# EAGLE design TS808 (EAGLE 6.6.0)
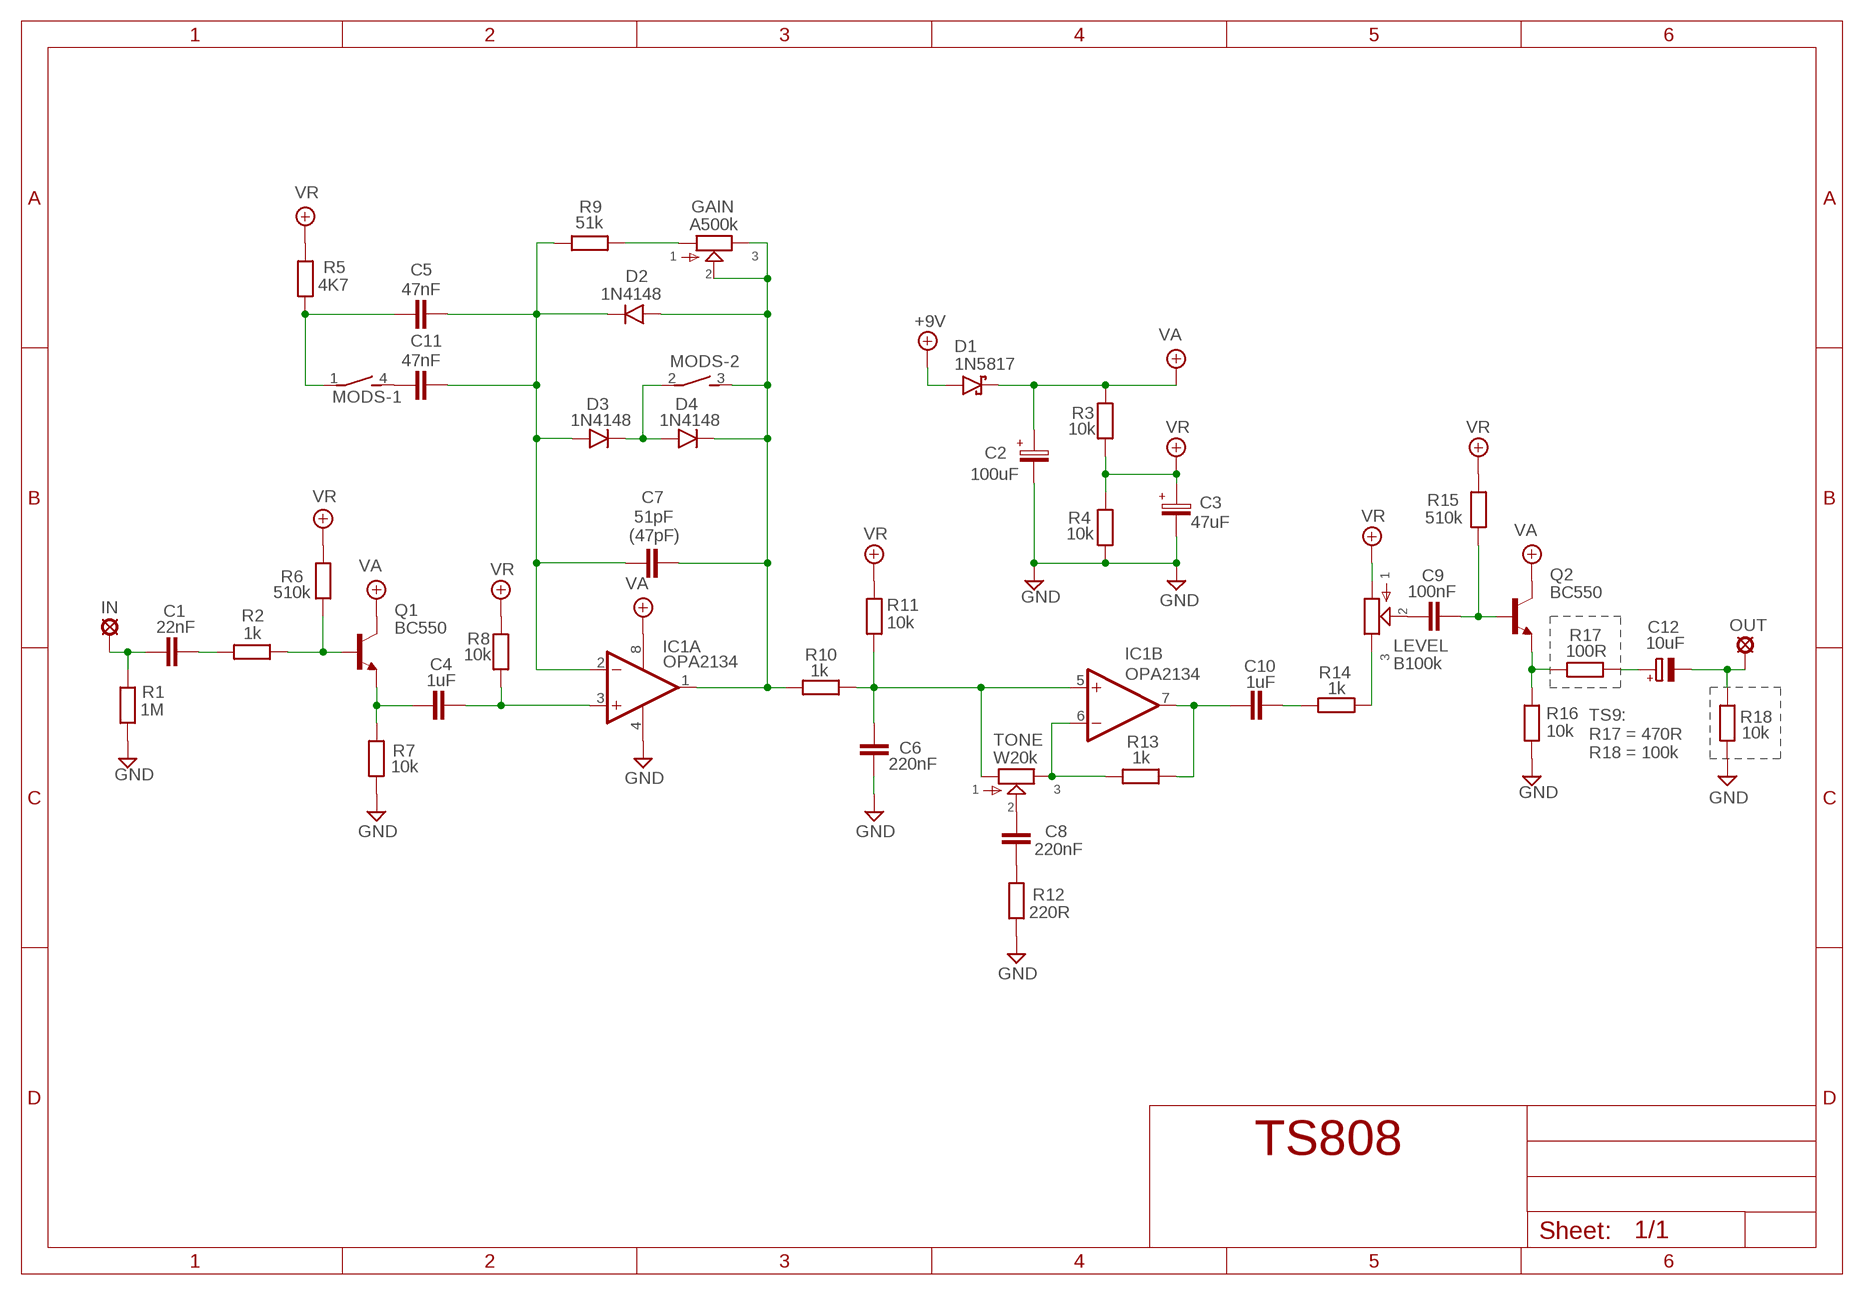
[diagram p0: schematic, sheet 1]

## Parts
+9V  +9V  +9V(T)1  [ROUND]
C1  22nF  22NF-82NF"  [4,5MM]
C2  100uF  063-EU  [063_025]
C3  47uF  063-EU  [063_025]
C4  1uF  072X0352  [072X035]
C5  47nF  22NF-82NF"  [4,5MM]
C6  220nF  100NF-220NF  [7,5MM]
C7  51pF  050X030_0251  [050X030_025]
C8  220nF  100NF-220NF  [7,5MM]
C9  100nF  100NF-220NF  [7,5MM]
C10  1uF  072X0352  [072X035]
C11  47nF  22NF-82NF"  [4,5MM]
C12  10uF  CPOL-EUE5-4  [E5-4]
D1  1N5817  [DO41-3]
D2  1N4148  1N4148-3  [DO35-3]
D3  1N4148  1N4148-3  [DO35-3]
D4  1N4148  1N4148-3  [DO35-3]
GAIN  A500k  POT-EU16MM  [16MM]
GND  GND  GND(T)1  [ROUND]
GND1  GND  GND(T)1  [ROUND]
IC1  OPA2134  LM4558N  [DIL08]
IN  MCS10B  [MCS10B]
LEVEL  B100k  POT-EU16MM  [16MM]
MODS  DS02E  [DS-02]
OUT  MCS10B  [MCS10B]
Q1  BC550  [TO92-]
Q2  BC550  [TO92-]
R1  1M  6MM-EU3  [R0207/3]
R2  1k  6MM-EU3  [R0207/3]
R3  10k  6MM-EU3  [R0207/3]
R4  10k  6MM-EU3  [R0207/3]
R5  4K7  6MM-EU3  [R0207/3]
R6  510k  6MM-EU3  [R0207/3]
R7  10k  6MM-EU3  [R0207/3]
R8  10k  6MM-EU3  [R0207/3]
R9  51k  6MM-EU3  [R0207/3]
R10  1k  6MM-EU3  [R0207/3]
R11  10k  6MM-EU3  [R0207/3]
R12  220R  6MM-EU3  [R0207/3]
R13  1k  6MM-EU3  [R0207/3]
R14  1k  6MM-EU3  [R0207/3]
R15  510k  6MM-EU3  [R0207/3]
R16  10k  6MM-EU3  [R0207/3]
R17  100R  6MM-EU3  [R0207/3]
R18  10k  6MM-EU3  [R0207/3]
TONE  W20k  POT-EU16MM  [16MM]

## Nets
+9V: +9V.1(+9V) D1.A
GND: C2.- C3.- C6.P$2 GND1.1(GND) GND.1(GND) IC1.4(P:V-) R1.1 R4.1 R7.1 R12.1 R16.1 R18.1
N$1: C8.P$1 TONE.2
N$2: C1.2 R2.1
N$3: Q1.2(B) R2.2 R6.1
N$4: C4.2 IC1.3(A:+IN) R8.1
N$5: C5.2 C7.1 C11.2 D2.C D3.A IC1.2(A:-IN) R9.1
N$6: C4.1 Q1.1(E) R7.2
N$7: C8.P$2 R12.2
N$8: GAIN.1 R9.2
N$9: C9.P$1 LEVEL.2
N$10: IC1.6(B:-IN) R13.1 TONE.3
N$11: C6.P$1 IC1.5(B:+IN) R10.2 R11.1 TONE.1
N$12: C11.1 MODS.4
N$13: D3.C D4.A MODS.2
N$14: C10.1 IC1.7(B:OUT) R13.2
N$15: C10.2 R14.1
N$16: LEVEL.3 R14.2
N$17: Q2.1(E) R16.2 R17.1
N$18: C1.1 IN.MP R1.2
N$19: C9.P$2 Q2.2(B) R15.1
N$20: C12.+ R17.2
N$21: C12.- OUT.MP R18.2
N$22: C7.2 D2.A D4.C GAIN.2 GAIN.3 IC1.1(A:OUT) MODS.3 R10.1
N$23: C5.1 MODS.1 R5.1
VA: C2.+ D1.C IC1.8(P:V+) Q1.3(C) Q2.3(C) R3.2
VR: C3.+ LEVEL.1 R3.1 R4.2 R5.2 R6.2 R8.2 R11.2 R15.2

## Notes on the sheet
- (47pF)
- TS9:
  R17 = 470R
  R18 = 100k

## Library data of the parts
+9V = gm-supply:+9V(T): +9V Voltage Supply
C1 C5 C11 = Mylar Kondensaattorit:22NF-82NF: 22nF-82nF
C2 C3 = Elektrolyytit:063-EU
C4 C10 = Wima MKS:072X035: 0.15 - 1.0uF;
C6 C8 C9 = Mylar Kondensaattorit:100NF-220NF: 100nF-220nF
C7 = Keraamiset kondensaattorit:050X030_025: 47 - 120pF
C12 = rcl:CPOL-EU: POLARIZED CAPACITOR, European symbol
D1 = Diodit:1N5817
D2-D4 = Diodit:1N4148: Fast Switching Diode
GAIN LEVEL TONE = gm-pots:POT-EU
GND GND1 = gm-supply:GND(T): Ground
IC1 = Operaatiovahvistimet:*4558: *4558 Op Amp Infamous for its use in tube screamers. This op amp has many manufacturers, hence the leading "*" in the name. The JRC4558 is a widely used example.
IN OUT = Padit:MCS10B: SOLDER PAD
MODS = switch-dil:DS02E: DIL/CODE SWITCH; OC_FARNELL: 9472126; OC_NEWARK: unknown
Q1 Q2 = Transistorit:BC550
R1-R18 = Vastukset:6MM-EU: 6mm Resistors (European schematic symbol)

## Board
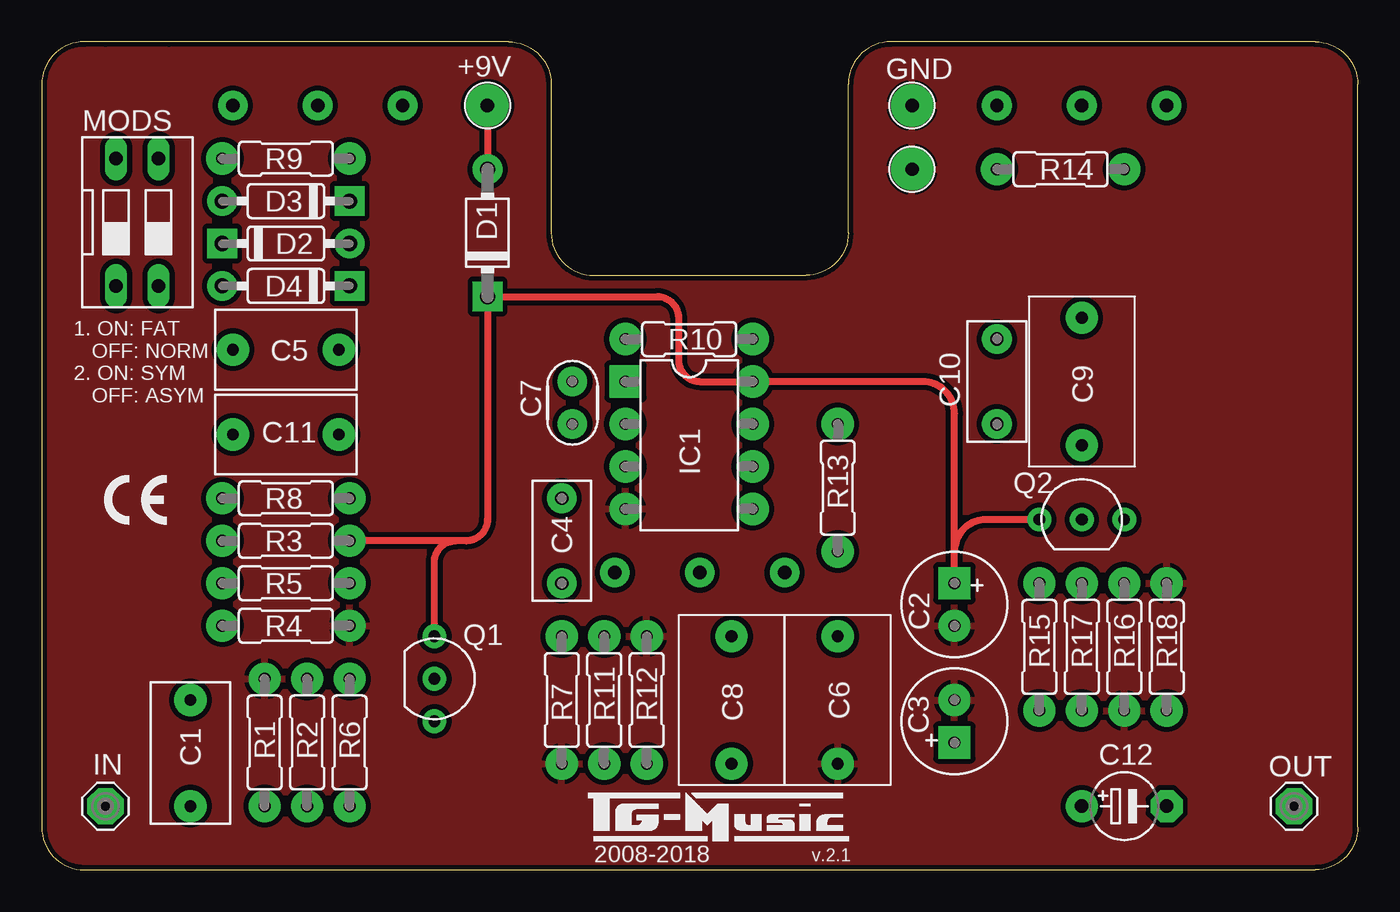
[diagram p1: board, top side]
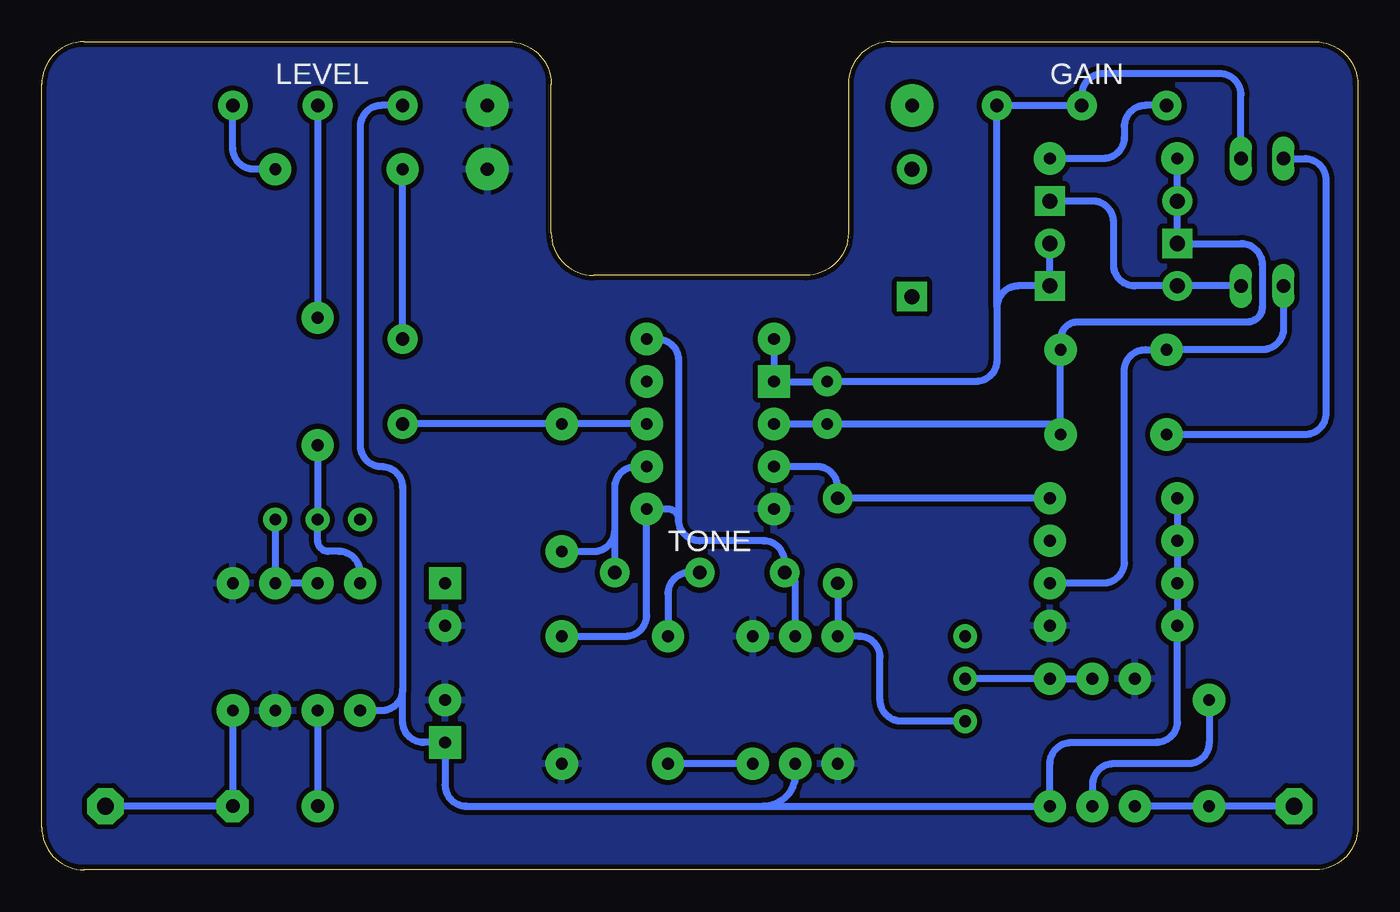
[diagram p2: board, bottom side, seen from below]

Size 78.74 x 49.53 mm. Coordinates in mm from the lower left corner, seen from the top.
Outline: 7.62,49.53 3.81,49.53
Outline: 78.74,2.54 78.74,46.99 arc90 76.2,49.53 50.8,49.53 arc90 48.26,46.99 48.26,38.1 arc-90 45.72,35.56 33.02,35.56 arc-90 30.48,38.1 30.48,46.99 arc90 27.94,49.53 2.54,49.53 arc90 0,46.99 0,2.54 arc90 2.54,0 76.2,0 arc90 78.74,2.54
Copper layers (1*16): Top 0.035mm / dielectric 1.5mm / Bottom 0.035mm
Design rules "ITEADstudio": minimum track width 10mil, minimum drill 12mil, track to track 12mil, track to pad 12mil, pad to pad 12mil, via to via 12mil, smd to smd 0mil, copper to edge 12mil, drill to drill 12mil, minimum pad ring 10mil, minimum via ring 6mil, stop-mask expansion 4mil, vias tented up to drill 100mil, thermal gap 10mil

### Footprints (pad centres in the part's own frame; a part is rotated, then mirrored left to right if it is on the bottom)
ROUND = drill 0.8 pad 2.54: 1 0,0
4,5MM = drill 0.7 pad 1.93: 1 -3.175,0; 2 3.175,0
063_025 = drill 0.7 pad 1.93 square: + -1.27,0 | drill 0.7 pad 1.93: - 1.27,0
072X035 = drill 0.8 pad 1.778: 1 -2.54,0; 2 2.54,0
7,5MM = drill 0.7 pad 1.93: P$1 -3.81,0; P$2 3.81,0
050X030_025 = drill 0.7 pad 1.778: 1 -1.27,0; 2 1.27,0
E5-4 = drill 0.813 pad 1.905: + -2.54,0 | drill 0.813 pad 1.905 octagon: - 2.54,0
DO41-3 = drill 0.9 pad 1.778: A 3.81,0 | drill 0.9 pad 1.778 square: C -3.81,0
DO35-3 = drill 0.9 pad 1.778: A 3.81,0 | drill 0.9 pad 1.778 square: C -3.81,0
16MM = drill 0.8 pad 1.778: 1 5.08,0; 2 0,0; 3 -5.08,0
DIL08 = drill 0.7 pad 1.93 square: 1 -3.81,-3.81 | drill 0.7 pad 1.93: 2 -1.27,-3.81; 3 1.27,-3.81; 4 3.81,-3.81; 5 3.81,3.81; 6 1.27,3.81; 7 -1.27,3.81; 8 -3.81,3.81
MCS10B = drill 1.016 pad 2.159 octagon: MP 0,0
DS-02 = drill 0.813 long: 1 -1.27,-3.81; 2 1.27,-3.81; 3 1.27,3.81; 4 -1.27,3.81
TO92- = drill 0.7 pad 1.422: 1 2.54,0; 2 0,0; 3 -2.54,0
R0207/3 = drill 0.7 pad 1.93: 1 -3.81,0; 2 3.81,0

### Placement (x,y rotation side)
+9V  26.67,45.72 0 top
C1  8.89,6.99 90 top
C2  54.61,15.88 270 top
C3  54.61,8.89 90 top
C4  31.11,19.68 90 top
C5  14.61,31.11 0 top
C6  47.62,10.16 270 top
C7  31.75,27.94 90 top
C8  41.27,10.16 270 top
C9  62.23,29.21 270 top
C10  57.15,29.21 90 top
C11  14.61,26.04 0 top
C12  64.77,3.81 0 top
D1  26.67,38.1 90 top
D2  14.61,37.47 0 top
D3  14.61,40.01 180 top
D4  14.61,34.92 180 top
GAIN  16.51,45.72 0 bottom
GND  52.07,45.72 0 top
GND1  52.07,41.91 0 top
IC1  38.73,25.4 270 top
IN  3.81,3.81 0 top
LEVEL  62.23,45.72 0 bottom
MODS  5.71,38.73 0 top
OUT  74.93,3.81 0 top
Q1  23.5,11.43 270 top
Q2  62.23,20.95 0 top
R1  13.34,7.62 270 top
R2  15.88,7.62 90 top
R3  14.61,19.68 0 top
R4  14.61,14.61 180 top
R5  14.61,17.14 180 top
R6  18.41,7.62 270 top
R7  31.11,10.16 90 top
R8  14.61,22.23 180 top
R9  14.61,42.55 0 top
R10  38.73,31.75 0 top
R11  33.66,10.16 270 top
R12  36.2,10.16 270 top
R13  47.62,22.86 90 top
R14  60.96,41.91 0 top
R15  59.69,13.34 270 top
R16  64.77,13.34 90 top
R17  62.23,13.34 270 top
R18  67.31,13.34 270 top
TONE  39.37,17.78 0 bottom

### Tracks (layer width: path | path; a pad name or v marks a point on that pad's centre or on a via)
+9V
  Top 0.406: +9V.1 D1.A
GND
  pour Bottom: 0,2.54 0,46.99 arc-90 2.54,49.53 27.94,49.53 arc-90 30.48,46.99 30.48,38.1 arc90 33.02,35.56 45.72,35.56 arc90 48.26,38.1 48.26,46.99 arc-90 50.8,49.53 76.2,49.53 arc-90 78.74,46.99 78.74,1.91 arc-90 76.83,0 2.54,0 arc-90
  pour Top: 0,2.54 0,46.99 arc-90 2.54,49.53 27.94,49.53 arc-90 30.48,46.99 30.48,38.1 arc90 33.02,35.56 45.72,35.56 arc90 48.26,38.1 48.26,46.99 arc-90 50.8,49.53 75.56,49.53 arc-90 78.74,46.35 78.74,2.54 arc-90 76.2,0 2.54,0 arc-90
N$1
  Bottom 0.406: TONE.2 40.01,17.78 arc-90 41.27,16.51 C8.P$1
N$2
  Bottom 0.406: C1.2 8.89,7.62 arc90 10.16,6.35 14.61,6.35 arc-90 15.88,5.08 R2.1
N$3
  Bottom 0.406: R2.2 R6.1 Q1.2
N$4
  Bottom 0.406: IC1.3 32.38,24.13 arc90 31.11,22.86 C4.2 R8.1
N$5
  Bottom 0.406: R9.1 D3.A D2.C 6.99,37.47 arc90 5.71,36.2 5.71,33.66 arc90 6.6,32.77 16.76,32.77 arc-90 17.78,31.75 C5.2 C11.2 arc-90 18.41,26.67 C7.1 IC1.2
N$6
  Bottom 0.406: C4.1 R7.2 29.84,13.97 arc90 28.57,12.7 28.57,10.16 arc-90 27.3,8.89 Q1.1
N$7
  Bottom 0.406: R12.2 C8.P$2
N$8
  Bottom 0.406: GAIN.1 12.7,45.72 arc-90 13.97,44.45 13.97,43.81 arc90 15.24,42.55 R9.2
N$9
  Bottom 0.406: LEVEL.2 C9.P$1
N$10
  Bottom 0.406: TONE.3 44.45,20.32 | 44.45,20.32 44.45,22.86 arc90 43.18,24.13 IC1.6 | R13.1 45.72,19.05 arc-90 44.45,20.32
N$11
  Bottom 0.406: R10.2 41.91,31.75 arc90 40.64,30.48 40.64,20.95 | R11.1 33.66,17.14 arc-90 TONE.1 34.29,18.41 arc-90 35.56,19.68 39.37,19.68 arc90 40.64,20.95 | C6.P$1 43.81,13.97 arc-90 42.55,15.24 IC1.5 41.27,21.59 arc90 40.64,20.95
N$12
  Bottom 0.406: MODS.4 3.17,42.55 arc90 1.91,41.27 1.91,27.3 arc90 3.17,26.04 C11.1
N$13
  Bottom 0.406: MODS.2 D4.A 13.34,34.92 arc90 14.61,36.2 14.61,38.73 arc-90 15.88,40.01 D3.C
N$14
  Bottom 0.406: IC1.7 R13.2 C10.1
N$15
  Bottom 0.406: C10.2 R14.1
N$16
  Bottom 0.406: R14.2 66.04,41.91 arc90 67.31,43.18 LEVEL.3
N$17
  Bottom 0.406: Q2.1 R16.2 R17.1
N$18
  Bottom 0.406: IN.MP C1.1 R1.2
N$19
  Bottom 0.406: C9.P$2 Q2.2 62.23,19.68 arc-90 61.59,19.05 60.96,19.05 arc90 59.69,17.78 R15.1
N$20
  Bottom 0.406: R17.2 C12.+
N$21
  Bottom 0.406: R18.2 C12.- OUT.MP
N$22
  Bottom 0.406: MODS.3 6.99,46.35 arc-90 8.26,47.62 15.24,47.62 arc-90 16.51,46.35 GAIN.2 GAIN.3 21.59,33.66 | D2.A D4.C 20.32,34.92 arc-90 21.59,33.66 | R10.1 IC1.1 C7.2 22.86,29.21 arc-90 21.59,30.48 21.59,33.66
N$23
  Bottom 0.406: MODS.1 4.45,32.38 arc90 5.71,31.11 C5.1 12.7,31.11 arc-90 13.97,29.84 13.97,18.41 arc90 15.24,17.14 R5.1
VA
  Top 0.406: C2.+ 54.61,19.05 | 54.61,19.05 54.61,27.3 arc90 52.7,29.21 IC1.8 39.37,29.21 arc-90 38.1,30.48 38.1,33.02 arc90 36.83,34.29 D1.C 26.67,20.95 arc-90 25.4,19.68 24.77,19.68 | Q2.3 56.52,20.95 arc90 54.61,19.05 | 24.77,19.68 R3.2 | Q1.3 23.5,18.41 arc-90 24.77,19.68
VR
  Bottom 0.406: R8.2 R3.1 R5.2 R4.2 10.79,8.89 arc90 12.06,7.62 17.14,7.62 arc-90 18.41,6.35 R6.2 35.56,3.81 | LEVEL.1 58.42,45.72 arc-90 59.69,44.45 59.69,25.4 arc-90 58.42,24.13 arc90 57.15,22.86 57.15,10.79 | 57.15,10.79 arc90 58.42,9.53 R15.2 | 35.56,3.81 53.34,3.81 arc90 54.61,5.08 C3.+ 55.88,7.62 arc90 57.15,8.89 57.15,10.79 | R11.2 33.66,5.71 arc90 35.56,3.81

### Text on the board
tNames: 1. ON: FAT / OFF: NORM / 2. ON: SYM / OFF: ASYM | 2008-2018 | v.2.1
